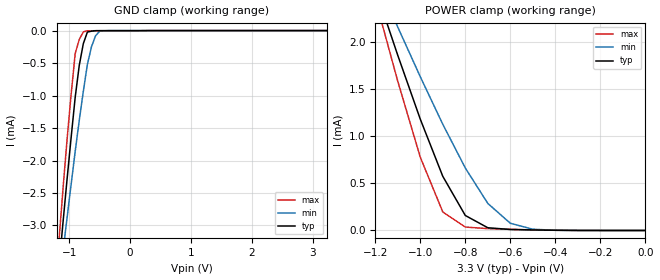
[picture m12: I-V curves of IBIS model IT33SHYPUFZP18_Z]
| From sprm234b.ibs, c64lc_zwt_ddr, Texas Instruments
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[Model]   IT33SHYPUFZP18_Z
Model_type   Input
Polarity   Non-Inverting
Vinl =  0.8V
Vinh =  2V
C_comp   0.7647563p   0.701391p   0.8403617p
[Model Spec]
Vinl   0.8V   0.8V   0.8V
Vinh   2V   2V   2V
[Temperature Range]   25   125   -40
[Voltage Range]   3.3   3.14   3.47
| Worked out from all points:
|   GND clamp passes 1 mA (typ) near -0.90 V on its own axis
|   POWER clamp passes 1 mA (typ) near -0.97 V on its own axis
[POWER_clamp]
|   voltage   I(typ)   I(min)   I(max)
-3.3V     17.7mA     14.37mA    20.92mA
-1.167V   2.338mA    2.525mA    2.173mA
-1.133V   2.101mA    2.344mA    1.88mA
-1.1V     1.864mA    2.164mA    1.588mA
-1.067V   1.637mA    1.988mA    1.319mA
-1V       1.184mA    1.636mA    779.8uA
-900mV    576uA      1.13mA     196.9uA
-800mV    159.5uA    664.7uA    36.48uA
-700mV    28.98uA    287.6uA    19.64uA
-600mV    10.75uA    76.67uA    12.02uA
-500mV    5.716uA    13.26uA    6.166uA
-11.55fV  96.05nA    92.8nA     223.3nA
[GND_clamp]
|   voltage   I(typ)   I(min)   I(max)
-3.3V     -26.08mA   -21.52mA   -29.08mA
-1.167V   -3.644mA   -3.938mA   -3.242mA
-1.1V     -2.956mA   -3.405mA   -2.438mA
-1.033V   -2.29mA    -2.882mA   -1.678mA
-900mV    -1.027mA   -1.86mA    -354.7uA
-833.3mV  -536.2uA   -1.383mA   -136.3uA
-766.7mV  -201.4uA   -936.8uA   -19.13uA
-700mV    -22.93uA   -521.4uA   -3.15uA
-633.3mV  -8.864uA   -252.1uA   -2.584uA
-566.7mV  -1.536uA   -81.8uA    -2.296uA
-500mV    -942.4nA   -10.4uA    -2.286uA
3.233V    94.43nA    99.21nA    210.7nA
